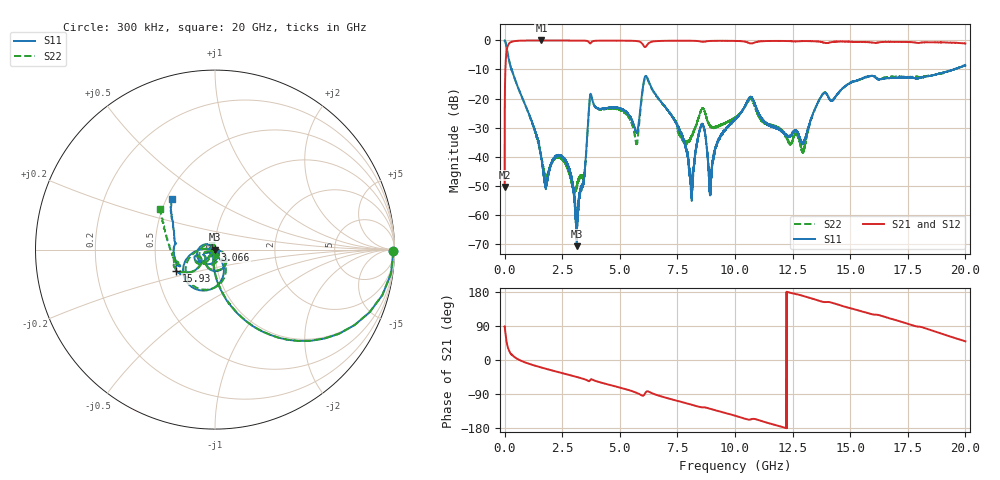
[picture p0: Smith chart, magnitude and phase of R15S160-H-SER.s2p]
!{R15S160}
!Johanson Technology Inc.
!www.johansontechnology.com
!Test Board Conditions:
!Substrate Type  RO4350B
!Substrate Thickness  20 mil
!Substrate Dk  3.66
!TL Type: GCPW
!TL Trace Width  34 mil
!TL Gap  10 mil
!Electrode orientation  Horizontal
!DUT TOPOLOGY	SERIES
!Mounting Pad LxW  26x52 mil
! Created Sat Feb  6 14:15:07 2021
# hz S ma R 50
! 2 Port Network Data from SP1.SP block
! freq  magS11  angS11  magS21  angS21  magS12  angS12  magS22  angS22
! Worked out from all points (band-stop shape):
!   20001 points, 300 kHz to 20 GHz, reference 50 ohm
!   highest |S21| = -0.01 dB at 1.596 GHz (marker M1); lowest = -50.5 dB at 300 kHz (marker M2)
!   |S21| within 3 dB of the highest: 99.91 MHz to end of sweep
!   lowest |S11| = -70.9 dB at 3.131 GHz (marker M3), VSWR 1.00, Z = 50 + j0.00347 ohm
!   |S11| at or under -10 dB: 289.5 MHz to 299.8 MHz (10.31 MHz wide, 3.5 % of centre); 309.6 MHz to 19.48 GHz (19.17 GHz wide, 194 % of centre); 19.48139 GHz to 19.48357 GHz (2.177 MHz wide, 0.0112 % of centre)
!   |S22| runs from -52.8 to 0.0 dB; largest |S21 - S12| = 0.016
!   S11 on the Smith chart (normalised r, x): 300 kHz: open; 3.066 GHz: 1.00, +0.00; 15.93 GHz: 0.63, -0.16; 20 GHz: 0.54, +0.35
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300000  0.9941 -0.3  0.002977 89.0  0.002944 89.9  0.9944 -0.3
1.023e8  0.6942 -47.2  0.7155 42.7  0.7165 42.6  0.6958 -47.0
1.763e8  0.4851 -63.0  0.8693 26.8  0.8698 26.7  0.4882 -62.7
1.5963e9  0.009142 -127.5  0.999 -19.9  0.9976 -19.8  0.00991 -85.1
2.6093e9  0.00875 70.4  0.9972 -36.4  0.9971 -36.4  0.007985 27.8
3.0663e9  0.0009849 84.5  0.9962 -43.7  0.9963 -43.7  0.002718 -60.6
3.1313e9  0.000286 173.0  0.9954 -44.8  0.9964 -44.8  0.003107 -81.6
3.3343e9  0.003018 -109.7  0.9943 -48.3  0.9945 -48.3  0.004488 -101.2
3.7593e9  0.1145 -104.3  0.9238 -50.7  0.9227 -50.7  0.1121 -103.2
5.7093e9  0.0263 -123.5  0.9785 -86.0  0.9783 -86.0  0.01705 -124.9
6.1063e9  0.2422 -110.6  0.7685 -87.2  0.77 -87.2  0.2317 -105.3
6.6673e9  0.1021 -176.4  0.9778 -93.6  0.9771 -93.6  0.09959 -175.1
8.1063e9  0.00216 85.7  0.9868 -117.9  0.9862 -117.8  0.02183 -101.4
8.5363e9  0.03516 -84.1  0.954 -124.9  0.9541 -124.9  0.06344 -97.1
8.9353e9  0.002787 57.3  0.9812 -129.0  0.9812 -129.0  0.0325 -117.6
1.00003e10  0.0432 -66.7  0.9819 -146.9  0.9818 -146.9  0.04666 -70.8
1.06953e10  0.1068 -153.7  0.8852 -156.5  0.8855 -156.5  0.09819 -142.2
1.29423e10  0.01655 176.7  0.9741 169.3  0.9748 169.3  0.01238 176.9
1.33343e10  0.04799 -132.0  0.9721 162.2  0.9726 162.2  0.04775 -121.1
1.59303e10  0.2456 -151.3  0.9214 121.1  0.9269 121.2  0.2447 -155.2
1.66673e10  0.2244 -159.7  0.9471 110.7  0.9362 110.6  0.2343 -160.0
2e10  0.3688 130.5  0.8878 49.2  0.8823 48.9  0.38 143.2
